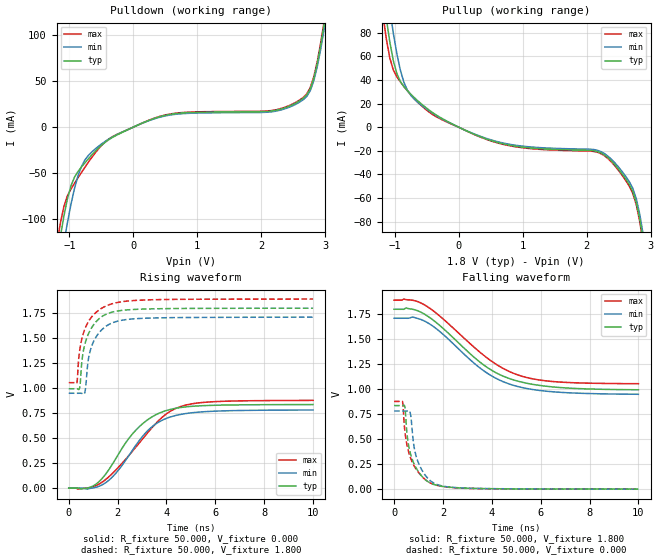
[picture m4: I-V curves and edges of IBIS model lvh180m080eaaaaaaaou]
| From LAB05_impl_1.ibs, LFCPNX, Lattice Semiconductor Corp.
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[Model] lvh180m080eaaaaaaaou
Model_type Output
Polarity   Non-Inverting
Enable   Active-High
Vmeas =  0.900V
Cref =  0.0F
Rref =  1.000M
Vref =  0.0V
C_comp   5.000pF   4.000pF   5.500pF
[Temperature Range]   25.000   0.125k   -40.000
[Voltage Range]   1.800V   1.710V   1.890V
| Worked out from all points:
|   slope of the pulldown table from 0 to 0.27 V, typ, clamps not added: 33.5 ohm
|   slope of the pullup table from 0 to 0.27 V, typ, clamps not added: 40.5 ohm
|   rising waveform, R_fixture 50.000, V_fixture 0.000: 20-80 % time 1.56ns typ, 1.52ns min, 1.89ns max; typ from 0 V to 0.836 V
|   rising waveform, R_fixture 50.000, V_fixture 1.800: 20-80 % time 531ps typ, 527ps min, 592ps max; typ from 0.994 V to 1.8 V
|   falling waveform, R_fixture 50.000, V_fixture 1.800: 20-80 % time 2.38ns typ, 2.27ns min, 2.45ns max; typ from 1.8 V to 0.994 V
|   falling waveform, R_fixture 50.000, V_fixture 0.000: 20-80 % time 525ps typ, 497ps min, 574ps max; typ from 0.836 V to 0 V
[Pulldown]
|Voltage   I(typ)   I(min)   I(max)
-1.8V     -455.8mA   -464.1mA   -455.9mA
-1.195V   -143.5mA   -173.1mA   -127.2mA
-1.085V   -96.8mA    -125.7mA   -86.3mA
-975mV    -63.89mA   -84mA      -67.31mA
-755mV    -38.62mA   -35.5mA    -43.42mA
-95mV     -3.13mA    -2.89mA    -2.938mA
565mV     13.74mA    13.05mA    14.15mA
2.16V     17.52mA    16.65mA    18.05mA
2.6V      28.66mA    27.23mA    29.52mA
2.82V     53mA       50.35mA    54.59mA
2.985V    113.1mA    107.4mA    116.5mA
3.6V      423.8mA    402.6mA    436.5mA
[Pullup]
|Voltage   I(typ)   I(min)   I(max)
-1.8V     423.8mA    442.4mA    413.3mA
-1.185V   114.8mA    145.2mA    96mA
-1.13V    92.1mA     121.8mA    74.8mA
-1.075V   72.1mA     99.6mA     58.48mA
-965mV    45.28mA    62.08mA    42.62mA
-800mV    30.91mA    31.23mA    30.7mA
-360mV    10.61mA    10.03mA    9.151mA
685mV     -14.03mA   -13.33mA   -14.45mA
2.225V    -21.86mA   -20.76mA   -22.51mA
2.665V    -48.46mA   -46.04mA   -49.91mA
2.885V    -96.4mA    -91.6mA    -99.3mA
3.6V      -453.8mA   -431.1mA   -467.4mA
[Ramp]
| variable   typ   min   max
dV/dt_r   0.649/1.570n   0.591/1.567n   0.606/1.928n
dV/dt_f   0.666/2.463n   0.624/2.370n   0.636/2.551n
R_load = 50.000
[Rising Waveform]
R_fixture = 50.000
V_fixture = 0.000
V_fixture_min = 0.000
V_fixture_max = 0.000
|  time   V(typ)   V(min)   V(max)
0s        109.1uV    -50.23uV   -498.6uV
899ps     11.2mV     -1.538mV   7.638mV
1.512ns   140.7mV    54.59mV    86.45mV
2.002ns   326.5mV    170.7mV    200.6mV
2.729ns   575.5mV    422.6mV    405.1mV
3.311ns   697.6mV    593.1mV    577.4mV
3.898ns   768.8mV    687.7mV    724.1mV
4.541ns   805.3mV    735.7mV    812.7mV
5.52ns    825.2mV    764mV      857.8mV
10ns      836.2mV    781.8mV    877.9mV
[Rising Waveform]
R_fixture = 50.000
V_fixture = 1.800
V_fixture_min = 1.710
V_fixture_max = 1.890
|  time   V(typ)   V(min)   V(max)
0s        994.1mV    949mV      1.055V
333ps     994.5mV    949.2mV    1.056V
431ps     991.7mV    949.3mV    1.347V
548ps     1.289V     946mV      1.504V
639ps     1.419V     945.7mV    1.578V
692ps     1.468V     1.008V     1.611V
798ps     1.539V     1.278V     1.663V
951ps     1.61V      1.428V     1.717V
1.709ns   1.756V     1.645V     1.839V
10ns      1.8V       1.71V      1.891V
[Falling Waveform]
R_fixture = 50.000
V_fixture = 1.800
V_fixture_min = 1.710
V_fixture_max = 1.890
|  time   V(typ)   V(min)   V(max)
0s        1.8V       1.71V      1.891V
502ps     1.812V     1.71V      1.896V
770ps     1.799V     1.722V     1.89V
1.298ns   1.743V     1.675V     1.836V
1.901ns   1.631V     1.571V     1.726V
3.68ns    1.24V      1.183V     1.337V
4.358ns   1.142V     1.086V     1.222V
5.09ns    1.079V     1.025V     1.141V
6.644ns   1.02V      971.4mV    1.074V
10ns      994.1mV    949mV      1.055V
[Falling Waveform]
R_fixture = 50.000
V_fixture = 0.000
V_fixture_min = 0.000
V_fixture_max = 0.000
|  time   V(typ)   V(min)   V(max)
0s        836.2mV    781.8mV    877.9mV
343ps     835.8mV    781.6mV    875.5mV
433ps     831.4mV    781.8mV    603.2mV
541ps     530.8mV    782.1mV    428.2mV
641ps     384.7mV    776.9mV    336.1mV
811ps     256.9mV    436.4mV    237.8mV
951ps     191.8mV    293.2mV    183.4mV
1.599ns   49.92mV    64.81mV    49.67mV
2.989ns   9.162mV    9.755mV    7.477mV
10ns      109.1uV    -50.23uV   -498.6uV
